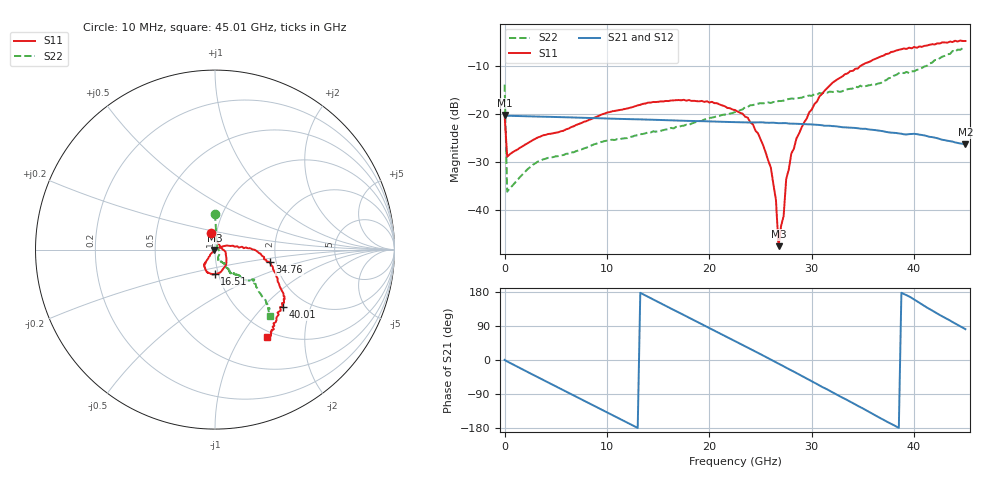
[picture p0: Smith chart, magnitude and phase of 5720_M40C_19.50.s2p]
! Device:  ADRF5720
! Description: 0.5dB LSB GaAs MMIC 6-bit Digital Attenuator
! Frequency:  0.000009 -  40 GHz
! Ports:
!	RF1	= Port 1
!	RF2	= Port 2
! Vdd:  3.3 Volt
! Vss:  -3.3 Volt
! Control:  0/3.3 Volt
! State:  19.50 dB attenuation
! Data:  The device was measured using G-S-G Probes on a matrix board.
!  Data was collected using an calibrated 4 port network analyzer.
!  The reference plane for this measurement is at the launchers.
! Note:  Analog Devices supplies this data as a sample of measured data
!  for this product.  Your particular data for this product may vary.
!  Data was taken at -40 degrees C.
!  Analog Devices reserves the right to change this data at anytime.
# GHZ S DB R 45.0
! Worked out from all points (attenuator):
!   181 points, 10 MHz to 45.01 GHz, reference 45 ohm
!   highest |S21| = -20.28 dB at 10 MHz (marker M1); lowest = -26.4 dB at 45.01 GHz (marker M2)
!   lowest |S11| = -47.6 dB at 26.76 GHz (marker M3), VSWR 1.01, Z = 44.7 - j0.205 ohm
!   |S11| at or under -10 dB: start of sweep to 34.82 GHz
!   |S22| runs from -36.3 to -6.3 dB; largest |S21 - S12| = 0.00039
!   S11 on the Smith chart (normalised r, x): 10 MHz: 0.94, +0.18; 16.51 GHz: 0.96, -0.27; 34.76 GHz: 1.85, -0.28; 40.01 GHz: 1.55, -1.30; 45.01 GHz: 0.91, -1.32
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0.01  -20.27 101.7  -20.28 0.3  -20.30 0.2  -13.97 90.3
0.26  -28.96 14.9  -20.45 -3.8  -20.47 -3.8  -36.26 32.2
3.26  -24.96 -9.5  -20.61 -45.5  -20.64 -45.5  -29.97 -32.0
7.76  -21.70 -39.3  -20.87 -107.3  -20.89 -107.3  -27.24 -65.4
15.26  -17.47 -82.9  -21.33 149.5  -21.35 149.5  -23.58 -68.2
16.51  -17.25 -90.7  -21.44 132.4  -21.46 132.3  -23.09 -65.2
20.26  -17.55 -110.6  -21.63 80.8  -21.66 80.7  -20.83 -57.9
22.76  -19.57 -125.8  -21.78 46.4  -21.80 46.4  -19.54 -58.1
24.26  -22.24 -127.1  -21.85 25.9  -21.87 25.8  -18.23 -56.8
26.01  -31.23 -133.6  -21.90 1.2  -21.92 1.1  -17.80 -56.0
26.51  -38.00 -126.0  -21.95 -6.2  -21.96 -6.3  -17.67 -57.1
26.76  -47.59 -146.7  -21.99 -9.6  -22.01 -9.7  -17.38 -55.4
27.01  -43.39 -23.3  -21.98 -13.0  -22.01 -13.1  -17.39 -56.9
27.26  -41.31 36.5  -21.99 -16.6  -22.01 -16.7  -17.30 -55.4
27.51  -33.61 14.9  -21.98 -20.3  -22.00 -20.4  -17.10 -56.6
28.01  -28.30 19.5  -22.08 -27.2  -22.11 -27.4  -16.87 -57.2
30.26  -18.05 8.8  -22.29 -59.7  -22.31 -59.8  -15.97 -56.5
32.01  -13.63 0.4  -22.60 -84.9  -22.62 -85.0  -15.48 -53.1
34.76  -10.07 -12.7  -23.14 -124.5  -23.17 -124.6  -14.19 -49.2
37.76  -7.18 -31.5  -23.96 -168.4  -23.98 -168.6  -12.55 -45.3
40.01  -6.12 -40.1  -24.21 159.6  -24.23 159.5  -11.19 -38.9
45.01  -4.89 -59.3  -26.35 81.3  -26.37 81.3  -6.33 -50.6
